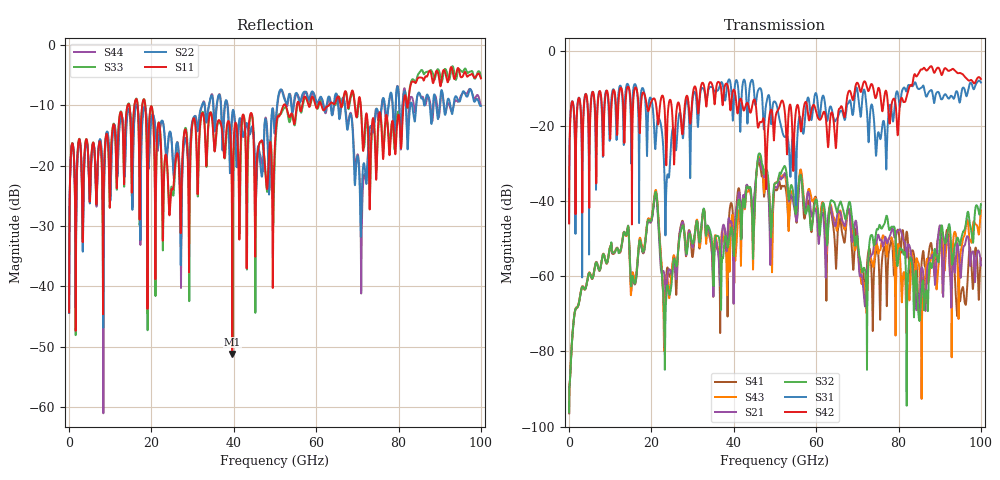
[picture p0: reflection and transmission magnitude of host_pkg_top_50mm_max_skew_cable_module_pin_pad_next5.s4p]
# Hz S RI R 50
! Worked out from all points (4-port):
!   10000 points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, 10 MHz to 100 GHz, reference 50 ohm
!   strongest paths, dB at 10 MHz, 25.01 GHz, 50.01 GHz, 75.01 GHz, 100 GHz:
!     S42: -45.9, -16.0, -18.9, -10.1, -7.5
!     S31: -45.8, -21.6, -13.5, -21.9, -8.4
!     S32: -96.2, -60.4, -35.2, -47.5, -40.8
!     S21: -96.4, -59.6, -36.2, -49.0, -57.1
!     S43: -96.4, -57.7, -35.2, -53.7, -42.5
!     S41: -96.5, -58.0, -36.9, -52.9, -55.2
!   lowest |S11| = -51.2 dB at 39.63 GHz (marker M1), VSWR 1.01, Z = 50.1 + j0.258 ohm
!   |S11| at or under -10 dB: start of sweep to 14.23 GHz; 18.48 GHz to 52.09 GHz (33.61 GHz wide, 95.2 % of centre); 70.83 GHz to 81.2 GHz (10.37 GHz wide, 13.6 % of centre)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
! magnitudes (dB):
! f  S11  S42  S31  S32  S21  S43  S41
! 10 MHz  -44.3  -45.9  -45.8  -96.2  -96.4  -96.4  -96.5
! 20.96 GHz  -38.9  -13.3  -26.0  -37.6  -38.3  -37.1  -37.8
! 23.24 GHz  -19.1  -16.2  -36.9  -84.8  -60.7  -67.5  -70.7
! 39.63 GHz  -51.2  -11.5  -15.8  -48.2  -48.2  -43.7  -41.6
! 46.26 GHz  -16.2  -19.1  -9.9  -27.3  -28.9  -28.3  -30.1
! 85.05 GHz  -5.4  -5.7  -10.1  -71.8  -71.1  -57.8  -67.1
! 100 GHz  -5.6  -7.5  -8.4  -40.8  -57.1  -42.5  -55.2
